(* Logix 5000 AddOnInstructionDefinition export; software revision 16.00 *)

ADD_ON_INSTRUCTION SCLP   (* revision 1.0, vendor Rockwell Automation *)
// Scale with Parameters
// Help:
// This routine performs the operation of the SLC-500 Scale With Parameters instruction (SCP).
// This output instruction consists of six parameters.  Parameters may be floating point or integer immediate data values or tags containing values.  The Input value is scaled to a range determined by creating a linear relationship between input min and max values and scaled min and max values.  The scaled result is returned to the tag indicated by the output parameter.
// The formula is as follows:
// Scaled value = (input value x rate) + offset
// Rate = (scaled max. - scaled min.) / (input max. - input min.)
// Offset = scaled minimum - (input minimum x rate)
// Note: The input minimum, input maximum, scaled minimum, and scaled maximum are used to determine the slope and offset values. The input value can go outside of the specified input limits and no ordering is required. For example, the scaled output value will not necessarily be clamped between the scaled minimum and scaled maximum values.
VAR_INPUT
   Input : REAL; {required}   // Value to be scaled
   InputMin : REAL; {required}   // Minimum value for the input (low end of range)
   InputMax : REAL; {required}   // Maximum value for the input (upper end of range)
   ScaledMin : REAL; {required}   // Minimum scaling value representing the low end of the linear range to which you want to scale the input
   ScaledMax : REAL; {required}   // Maximum scaling value representing the upper end of the linear range to which you want to scale the input
END_VAR
VAR_OUTPUT
   Output : REAL; {required}   // Resulting scaled value that is returned after the instruction is executed
END_VAR
VAR
   Temp1 : REAL;
   Temp2 : REAL;
   Rate : REAL;
   Temp4 : REAL;
   Offset : REAL;
   Temp3 : REAL;
END_VAR

ROUTINE Logic   (* ladder *)
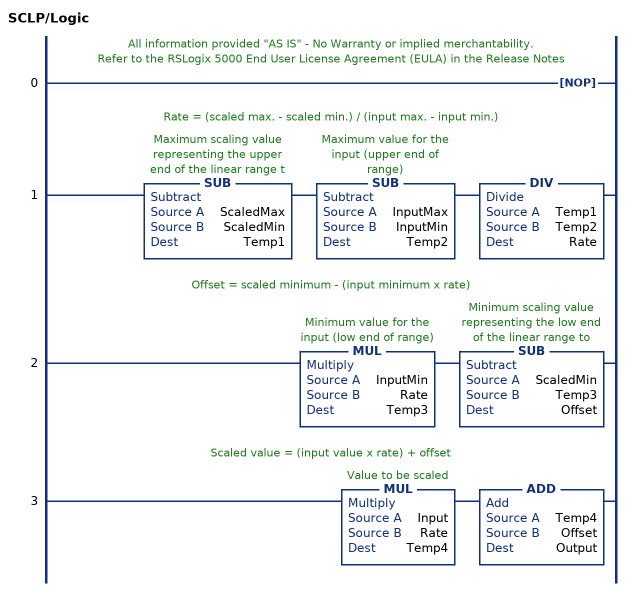
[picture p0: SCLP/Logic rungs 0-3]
   // All information provided "AS IS" - No Warranty or implied merchantability.
   // Refer to the RSLogix 5000 End User License Agreement (EULA) in the Release Notes
   0: NOP();
   // Rate = (scaled max. - scaled min.) / (input max. - input min.)
   1: SUB(ScaledMax,ScaledMin,Temp1)SUB(InputMax,InputMin,Temp2)DIV(Temp1,Temp2,Rate);
   // Offset = scaled minimum - (input minimum x rate)
   2: MUL(InputMin,Rate,Temp3)SUB(ScaledMin,Temp3,Offset);
   // Scaled value = (input value x rate) + offset
   3: MUL(Input,Rate,Temp4)ADD(Temp4,Offset,Output);
END_ROUTINE
END_ADD_ON_INSTRUCTION
